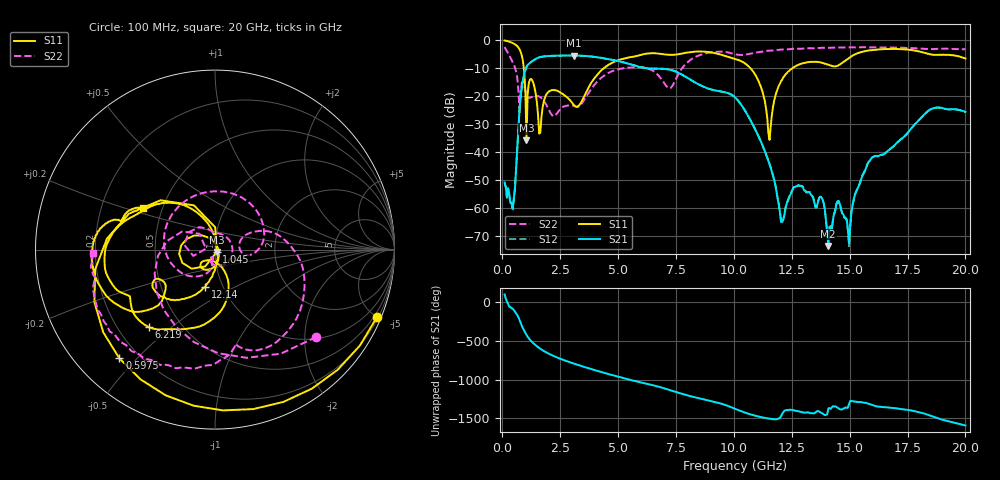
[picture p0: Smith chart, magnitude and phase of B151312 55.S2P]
!  2-Port S-parameters saved by WinCal
! VAR MeasName=S-Parameters (CALIBRATED_DATA) read from VNA (N5244A)
! VAR MeasDate=12/8/2015 5:48:04 PM
! VAR NAME=B151312 55
! VAR FILENAME=B151312 55.S2P
! VAR DATE=12/8/2015 5:48:05 PM
! VAR PHYS_PORTS=1,2
# Hz S DB R 50
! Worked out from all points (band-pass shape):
!   401 points, 100 MHz to 20 GHz, reference 50 ohm
!   highest |S21| = -5.58 dB at 3.085 GHz (marker M1); lowest = -73.6 dB at 14.08 GHz (marker M2)
!   |S21| within 3 dB of the highest: 1.145 GHz to 5.476 GHz (4.331 GHz wide, 131 % of centre)
!   lowest |S11| = -35.8 dB at 1.045 GHz (marker M3), VSWR 1.03, Z = 51 - j1.33 ohm
!   |S11| at or under -10 dB: 927.6 MHz to 4.399 GHz (3.472 GHz wide, 130 % of centre); 10.7 GHz to 12.55 GHz (1.842 GHz wide, 15.8 % of centre)
!   |S22| runs from -27.2 to -2.6 dB; largest |S21 - S12| = 0.0019
!   S11 on the Smith chart (normalised r, x): 100 MHz: 0.29, -4.99; 597.5 MHz: 0.13, -0.45; 1.045 GHz: 1.02, -0.03; 6.219 GHz: 0.33, -0.42; 12.14 GHz: 0.82, -0.36; 20 GHz: 0.39, +0.23
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1e8  -0.20 -22.6  -50.93 98.2  -51.16 96.8  -2.55 -40.8
4.4825e8  -1.13 -97.9  -60.12 -83.8  -60.56 -82.0  -7.95 -144.2
5.975e8  -1.86 -131.3  -45.83 -144.4  -45.81 -145.1  -11.34 169.7
1.04525e9  -35.81 -53.5  -9.68 -62.8  -9.68 -62.8  -19.76 100.0
1.3935e9  -17.07 146.2  -7.03 175.9  -7.03 175.9  -20.20 -0.3
1.5925e9  -33.49 61.7  -6.25 128.8  -6.25 128.8  -20.23 -59.2
1.84125e9  -20.60 -91.2  -5.85 81.2  -5.85 81.3  -22.38 -105.1
3.085e9  -23.21 -122.1  -5.58 -72.2  -5.58 -72.2  -23.57 -114.4
3.43325e9  -21.87 -78.7  -5.67 -106.0  -5.67 -106.0  -22.77 -103.9
4.9755e9  -7.32 -100.1  -7.51 120.4  -7.51 120.4  -10.52 160.2
6.21925e9  -4.92 -130.4  -10.08 28.1  -10.07 28.0  -10.07 38.9
6.7665e9  -4.91 -144.7  -10.27 -12.5  -10.27 -12.7  -12.93 -3.8
1.005e10  -6.79 151.9  -20.50 64.5  -20.51 64.3  -5.12 -76.4
1.15425e10  -35.72 -7.5  -44.33 -63.3  -44.34 -63.6  -3.83 -91.9
1.21395e10  -13.34 -105.1  -63.91 21.9  -64.19 25.2  -3.42 -101.0
1.338325e10  -7.82 -144.5  -55.82 7.2  -55.74 7.3  -2.99 -117.6
1.407975e10  -8.81 -153.4  -73.63 67.1  -73.19 65.6  -2.83 -126.4
1.45275e10  -9.01 -141.0  -57.50 70.4  -58.04 70.7  -2.75 -130.9
1.497525e10  -6.48 -136.5  -72.52 126.9  -73.69 139.7  -2.66 -135.8
1.5821e10  -3.76 -154.7  -43.62 127.5  -43.65 126.6  -2.65 -144.8
1.67165e10  -3.27 -172.0  -39.30 79.1  -39.23 78.5  -2.69 -152.9
2e10  -6.63 150.0  -25.71 -150.9  -25.83 -151.2  -3.33 -178.5
